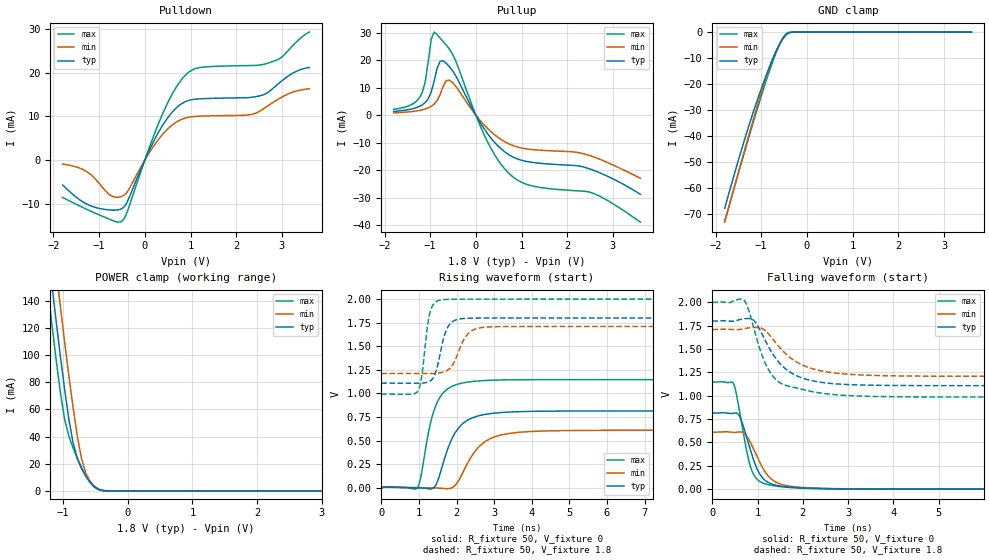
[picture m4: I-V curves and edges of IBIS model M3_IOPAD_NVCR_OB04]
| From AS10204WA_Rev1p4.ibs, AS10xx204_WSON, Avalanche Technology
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[Model] M3_IOPAD_NVCR_OB04
Model_type I/O
Enable   Active-High
Vinl  =  0.54
Vinh  =  1.26
Vmeas =  0.9
Cref  =  30e-12
| Capacitance  typ   min   max
C_comp   3.869840e-12   3.575244e-12   4.208825e-12
| Variables   typ   min   max
[GND Clamp Reference]   0   0   0
[POWER Clamp Reference]   1.8   1.71   2
[Pulldown Reference]   0   0   0
[Pullup Reference]   1.8   1.71   2
[Temperature Range]   25   105   -40
[Voltage Range]   1.8   1.71   2
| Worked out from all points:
|   slope of the pulldown table from 0 to 0.27 V, typ, clamps not added: 46.6 ohm
|   slope of the pullup table from 0 to 0.27 V, typ, clamps not added: 38.6 ohm
|   GND clamp passes 1 mA (typ) near -0.46 V on its own axis
|   POWER clamp passes 1 mA (typ) near -0.44 V on its own axis
|   falling waveform, R_fixture 50, V_fixture 0: 20-80 % time 347ps typ, 419ps min, 280ps max; typ from 0.814 V to 0 V
|   falling waveform, R_fixture 50, V_fixture 1.8: 20-80 % time 649ps typ, 769ps min, 500ps max; typ from 1.8 V to 1.1 V
|   rising waveform, R_fixture 50, V_fixture 0: 20-80 % time 520ps typ, 636ps min, 397ps max; typ from 0 V to 0.814 V
|   rising waveform, R_fixture 50, V_fixture 1.8: 20-80 % time 256ps typ, 352ps min, 184ps max; typ from 1.1 V to 1.8 V
[GND Clamp]
| Voltage   I(typ)   I(min)   I(max)
-1.8V     -67.84mA   -73.19mA   -72.81mA
-1.499V   -49.26mA   -53.93mA   -54.28mA
-1.303V   -37.87mA   -41.64mA   -42.4mA
-1.108V   -27.29mA   -29.68mA   -30.84mA
-912.4mV  -17.6mA    -18.46mA   -19.84mA
-782.1mV  -11.7mA    -11.87mA   -13.01mA
-651.7mV  -6.447mA   -6.494mA   -6.896mA
-521.4mV  -2.255mA   -2.526mA   -2.141mA
-456.2mV  -849.3uA   -1.156mA   -679.4uA
-391mV    -172uA     -356.5uA   -88.88uA
-260.7mV  -2.088uA   -12.98uA   -254.3nA
3.6V      0A         0A         0A
[POWER Clamp]
| Voltage   I(typ)   I(min)   I(max)
-1.8V     419.8mA    456.6mA    390.9mA
-1.238V   178mA      215.7mA    148.4mA
-1.173V   151mA      188.6mA    121.7mA
-1.108V   124.5mA    161.8mA    96mA
-1.043V   98.85mA    135.4mA    72.14mA
-977.6mV  74.56mA    109.6mA    52.56mA
-912.4mV  52.76mA    84.78mA    40.16mA
-847.2mV  35.48mA    61.36mA    31.71mA
-716.9mV  16.42mA    23.91mA    17.31mA
-651.7mV  10.9mA     13.27mA    11.28mA
-456.2mV  1.168mA    1.554mA    921.1uA
3.6V      0A         0A         0A
[Pulldown]
| Voltage   I(typ)   I(min)   I(max)
-1.8V     -5.69mA    -910.5uA   -8.548mA
-1.173V   -10.5mA    -3.41mA    -11.73mA
-782.1mV  -11.39mA   -7.821mA   -13.47mA
-521.4mV  -11.21mA   -8.363mA   -14.11mA
-391mV    -9.672mA   -7.354mA   -11.98mA
372.4mV   7.658mA    5.676mA    10.17mA
869mV     13.26mA    9.551mA    19.2mA
1.241V    14.01mA    10.05mA    21.19mA
2.352V    14.36mA    10.46mA    21.6mA
2.766V    16.04mA    12.9mA     22.39mA
3.248V    19.92mA    15.56mA    26.27mA
3.6V      21.15mA    16.29mA    29.24mA
[Pullup]
| Voltage   I(typ)   I(min)   I(max)
-1.8V     1.352mA    850uA      2.099mA
-1.238V   3.177mA    1.737mA    6.26mA
-1.108V   4.622mA    2.263mA    12.15mA
-977.6mV  8.411mA    3.225mA    27.68mA
-912.4mV  12.48mA    4.062mA    30.16mA
-782.1mV  19.57mA    7.55mA     27.92mA
-586.6mV  17.73mA    12.75mA    24.14mA
248.3mV   -6.519mA   -4.68mA    -9.425mA
744.8mV   -14.56mA   -10.55mA   -21.44mA
1.241V    -17.12mA   -12.46mA   -25.69mA
2.559V    -19.89mA   -15mA      -28.27mA
3.6V      -28.69mA   -22.89mA   -38.81mA
[Ramp]
dV/dt_r   0.488568/0.519945n  0.365787/0.635811n  0.687926/0.397312n
dV/dt_f   0.417076/0.649039n  0.300973/0.768787n  0.608145/0.500349n
R_load = 50
[Falling Waveform]
R_fixture = 50
V_fixture = 0
V_fixture_min = 0
V_fixture_max = 0
| Time   V(typ)   V(min)   V(max)
0s        814.3mV    609.6mV    1.147V
474.1ps   813.8mV    607.7mV    1.125V
599.7ps   783.2mV    612.6mV    837.3mV
776.9ps   525.9mV    556.8mV    365.8mV
948.2ps   264.1mV    391.6mV    129.1mV
1.058ns   153.3mV    278.2mV    80.21mV
1.23ns    73.11mV    143.7mV    48.66mV
1.546ns   30.54mV    48.34mV    24.51mV
3.663ns   898uV      1.414mV    777.2uV
21.88ns   242.1nV    617.1nV    249.8nV
[Falling Waveform]
R_fixture = 50
V_fixture = 1.8
V_fixture_min = 1.71
V_fixture_max = 2
| Time   V(typ)   V(min)   V(max)
0s        1.8V       1.71V      2V
684.9ps   1.824V     1.718V     2.031V
791.9ps   1.828V     1.727V     1.935V
954.3ps   1.787V     1.732V     1.656V
1.128ns   1.633V     1.714V     1.397V
1.355ns   1.433V     1.596V     1.2V
1.831ns   1.222V     1.372V     1.089V
2.549ns   1.136V     1.255V     1.02V
4.579ns   1.109V     1.211V     987.9mV
21.88ns   1.105V     1.208V     986.4mV
[Rising Waveform]
R_fixture = 50
V_fixture = 0
V_fixture_min = 0
V_fixture_max = 0
| Time   V(typ)   V(min)   V(max)
0s        74.44nV    376.1nV    131.9nV
944.2ps   468.1uV    1.945mV    -6.144mV
1.049ns   -1.961mV   1.585mV    113mV
1.314ns   -12.28mV   -657.4uV   697.4mV
1.509ns   84.57mV    -3.643mV   925.6mV
1.949ns   574.2mV    19.61mV    1.087V
2.418ns   740.7mV    345.5mV    1.126V
3.037ns   792.2mV    543.4mV    1.141V
4.152ns   810.9mV    599.7mV    1.146V
21.88ns   814.3mV    609.6mV    1.147V
[Rising Waveform]
R_fixture = 50
V_fixture = 1.8
V_fixture_min = 1.71
V_fixture_max = 2
| Time   V(typ)   V(min)   V(max)
0s        1.105V     1.208V     986.4mV
973.3ps   1.108V     1.21V      1.024V
1.065ns   1.109V     1.21V      1.158V
1.296ns   1.131V     1.21V      1.861V
1.443ns   1.219V     1.212V     1.968V
1.614ns   1.514V     1.223V     1.992V
1.902ns   1.764V     1.306V     1.998V
2.276ns   1.796V     1.619V     1.999V
2.814ns   1.799V     1.704V     1.999V
21.88ns   1.8V       1.71V      2V
